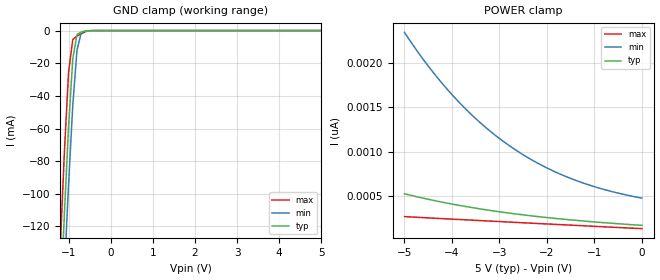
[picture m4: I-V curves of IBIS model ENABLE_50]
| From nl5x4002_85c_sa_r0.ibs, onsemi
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[Model]   ENABLE_50
Model_type Input
Vinh=3.5
Vinl=1.5
C_comp   4.0p   NA   NA
[Model Spec]
Vinh   3.5   3.15   3.85
Vinl   1.5   1.35   1.65
[Temperature Range] 25   85   -40
[Voltage Range]   5.0   4.5   5.5
[Pullup Reference]  5.0   4.5   5.5
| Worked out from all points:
|   GND clamp passes 1 mA (typ) near -0.71 V on its own axis
[GND Clamp]
-5V       -2.672A    -2.629A    -2.72A
-1.2V     -171.7mA   -206.9mA   -134.3mA
-1.1V     -112.8mA   -149mA     -74.83mA
-1V       -58.71mA   -94.21mA   -25.39mA
-900mV    -17.28mA   -45.7mA    -5.488mA
-800mV    -2.447mA   -11.99mA   -3.347mA
-700mV    -836.3uA   -1.356mA   -2.02mA
-600mV    -357.3uA   -195.6uA   -652.3uA
-400mV    -8.492uA   -9.966uA   -5.196uA
5V        167.7pA    475.1pA    130.8pA
[POWER Clamp]
-5V       524.3pA    2.344nA    266.6pA
-4.8V     498.4pA    2.185nA    260.8pA
-4.5V     462.2pA    1.964nA    252.3pA
-4.2V     429pA      1.765nA    243.8pA
-3.9V     398.4pA    1.584nA    235.4pA
-3.4V     353pA      1.323nA    221.6pA
-3.1V     328.8pA    1.189nA    213.3pA
-2.8V     306.6pA    1.069nA    205.2pA
-2.2V     267.6pA    870.7pA    189pA
-1.5V     229.8pA    697.2pA    170.3pA
-800mV    198.3pA    573.1pA    151.8pA
0V        167.7pA    475.1pA    130.8pA
